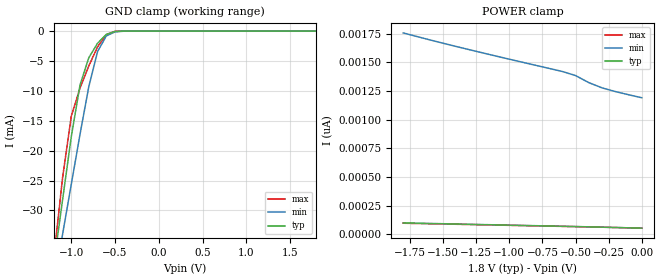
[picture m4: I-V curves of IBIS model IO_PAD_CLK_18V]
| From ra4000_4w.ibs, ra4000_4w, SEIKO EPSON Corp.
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[Model]   IO_PAD_CLK_18V
Model_type Input
Polarity Non-Inverting
Vinh=1.26
Vinl=0.54
C_comp   2.5p   2.0p   3.0p
[Temperature Range] 25   125   -40
[Voltage Range]   1.80   1.60   2.00
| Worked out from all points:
|   GND clamp passes 1 mA (typ) near -0.63 V on its own axis
[GND Clamp]
-1.8V     -103.9mA   -93.29mA   -119.4mA
-1.2V     -38.93mA   -42.41mA   -37.91mA
-1.1V     -28.21mA   -33.99mA   -24.53mA
-1V       -17.61mA   -25.59mA   -14.2mA
-900mV    -8.983mA   -17.21mA   -9.508mA
-800mV    -4.448mA   -9.271mA   -5.815mA
-700mV    -2.032mA   -3.421mA   -2.638mA
-600mV    -545.3uA   -803.9uA   -605.9uA
-500mV    -56.89uA   -135.5uA   -35.53uA
-400mV    -3.147uA   -16.88uA   -734nA
1.8V      53.93pA    1.246nA    48.52pA
[POWER Clamp]
-1.8V     100pA      1.758nA    97.1pA
-1.6V     95.05pA    1.697nA    92.5pA
-1.3V     87.65pA    1.611nA    85.6pA
-600mV    70.49pA    1.421nA    69.48pA
-500mV    68.04pA    1.386nA    67.18pA
-400mV    65.44pA    1.324nA    64.86pA
-300mV    62.59pA    1.278nA    62.26pA
-200mV    59.7pA     1.246nA    59.52pA
0V        53.93pA    1.192nA    54.02pA
